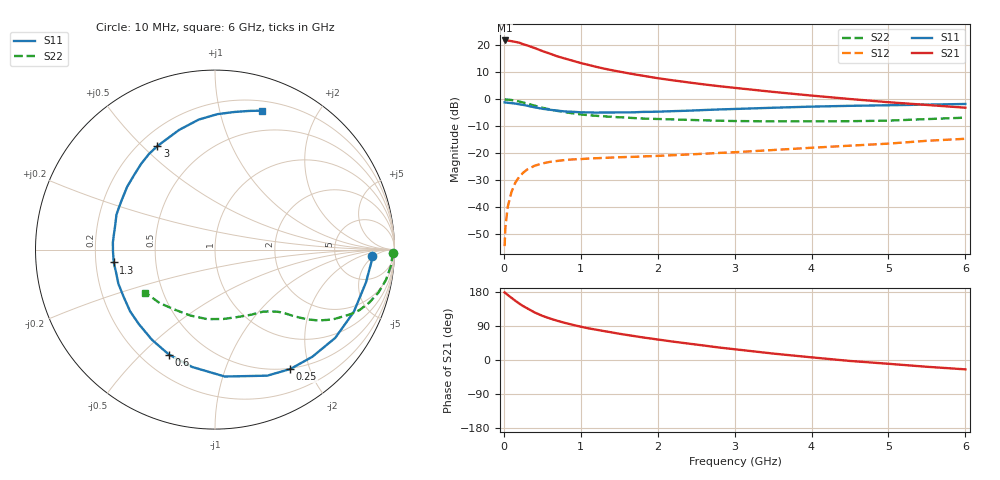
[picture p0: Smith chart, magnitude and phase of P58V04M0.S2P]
! SIEMENS Small Signal Semiconductors
! BFP183
! Si NPN RF Bipolar Junction Transistor in SOT143
! VCE = 8 V  IC = 4 mA
! Common Emitter S-Parameters:  March  1996
# GHz  S  MA  R  50
!  f  S11  S21  S12  S22
! GHz  MAG  ANG  MAG  ANG  MAG  ANG  MAG  ANG
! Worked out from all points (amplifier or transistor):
!   36 points, 10 MHz to 6 GHz, reference 50 ohm
!   highest |S21| = 21.8 dB at 10 MHz (marker M1)
!   |S21| within 3 dB of that: start of sweep to 418.2 MHz
!   unconditionally stable (mu >= 1): 1.804 GHz to 5.755 GHz
!   at 250 MHz: K = 0.17, MSG = 23.8 dB, |S12| = -27.3 dB
!   at 1.4 GHz: K = 0.84, MSG = 16.2 dB, |S12| = -21.6 dB
!   at 6 GHz: K = 0.96, MSG = 5.8 dB, |S12| = -14.6 dB
!   S11 on the Smith chart (normalised r, x): 10 MHz: 14, -4; 250 MHz: 0.49, -1.71; 600 MHz: 0.31, -0.61; 1.3 GHz: 0.28, -0.06; 3 GHz: 0.27, +0.56; 6 GHz: 0.29, +1.35
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0.01  0.8751 -2.4  12.27 178.3  0.0019 86.2  0.9941 -1.0
0.02  0.8736 -4.7  12.23 177.1  0.0042 84.2  0.989 -2.1
0.05  0.8607 -12.3  12.26 171.7  0.0101 86.0  0.9851 -5.1
0.15  0.8311 -36.3  11.54 156.2  0.0287 70.8  0.9417 -14.7
0.2  0.8065 -47.8  11.15 149.0  0.0366 66.0  0.9085 -19.0
0.25  0.7864 -57.8  10.47 142.4  0.0434 60.0  0.8718 -22.8
0.3  0.7603 -67.5  9.966 136.8  0.0496 55.9  0.8335 -25.7
0.4  0.7092 -85.6  8.892 125.5  0.0587 48.2  0.7612 -30.8
0.5  0.6662 -101.0  7.82 116.6  0.0647 42.2  0.6973 -34.5
0.6  0.6386 -113.7  6.982 109.5  0.0692 38.0  0.6476 -36.9
0.7  0.6129 -125.0  6.198 103.2  0.0722 34.8  0.6064 -38.7
0.8  0.5936 -135.5  5.643 97.6  0.075 32.2  0.5744 -40.2
0.9  0.5849 -143.9  5.146 92.6  0.0769 30.5  0.5462 -41.4
1.1  0.571 -160.5  4.324 83.6  0.0797 28.1  0.5066 -43.6
1.3  0.5688 -172.8  3.697 76.4  0.082 26.3  0.482 -45.7
1.7  0.5733 165.4  2.885 63.0  0.0858 25.6  0.4474 -50.5
2.2  0.6018 144.4  2.239 48.5  0.0919 26.0  0.4222 -57.5
3  0.6602 119.1  1.626 28.4  0.1044 27.1  0.3949 -72.4
3.5  0.6961 106.7  1.368 17.0  0.1147 27.4  0.3894 -83.4
4.5  0.755 88.9  1.01 -2.5  0.1381 25.4  0.3922 -110.3
5.5  0.7951 76.3  0.784 -17.9  0.17 22.1  0.4289 -136.0
6  0.8174 71.3  0.697 -24.7  0.1852 18.5  0.4561 -148.3
